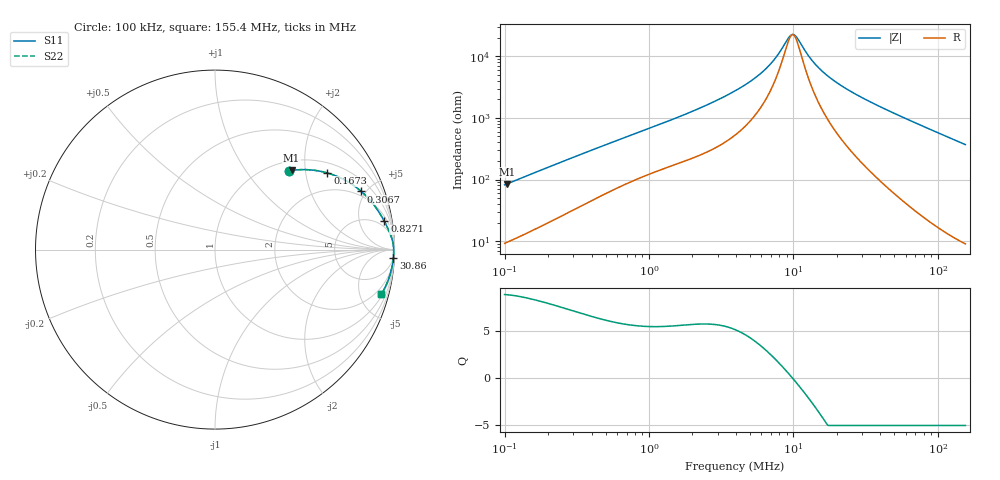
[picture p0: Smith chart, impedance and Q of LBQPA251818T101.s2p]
! LBQPA251818T101  S-PARAMETER MODEL  ( General Type )
! Model Generated by TAIYO YUDEN Corporation (http://www.ty-top.com)
! Version 1.0
! TAIYO YUDEN Control No. 191025NI43SB-FBB
! Copyright(c) 2019 TAIYO YUDEN CO.,LTD. All Rights Reserved.
! Product Description (link to TY-COMPAS)
! https://ds.yuden.co.jp/TYCOMPAS/or/detail?pn=LBQPA251818T101K&u=M
! Products Name : Inductors
! Characteristics :
!  Inductance : 100 uH , SRF(min) : 9.0 MHz , DC Resistance(max) : 4.81 Ohm
!  Rated Current : Saturation :160 mA , Temp Rise : 125 mA (20 degC)
!  Case Size : 2.5 x 1.8 / 0.098 x 0.071 [mm/inch] , Thickness : 1.8 / 0.071 [mm/inch]
!  (Conditions: Temperature = 25 degC , DC Bias Current/Voltage = 0A / 0V)
! External Node Assignments :
!  1  o---GGG---o  2
! GND o---------o GND
! Frequency Range : 0.1MHz  -  155.401204MHz  [ 402 STEP ]
# MHz S RI R 50
! Freq[MHz].  S11 Real  S11 Imag  S21 Real  S21 Imag  S12 Real  S12 Imag  S22 Real  S22 Imag
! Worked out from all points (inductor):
!   401 points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, 100 kHz to 155.4 MHz, reference 50 ohm
!   read as one part in series: L = 128 uH near 103.7 kHz
!   highest Q = 8.83 at 103.7 kHz (marker M1), where L = 129 uH
!   self-resonance near 9.698 MHz
!   S11 on the Smith chart (normalised r, x): 100 kHz: 1.18, +1.63; 167.3 kHz: 1.32, +2.65; 306.7 kHz: 1.66, +4.65; 827.1 kHz: 3, +11; 30.86 MHz: 4, -41; 155.4 MHz: 1.18, -7.37
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0.1  0.4112 0.4388  0.5888 -0.4388  0.5888 -0.4388  0.4112 0.4388
0.103743  0.4267 0.4412  0.5733 -0.4412  0.5733 -0.4412  0.4267 0.4412
0.167264  0.6261 0.4269  0.3739 -0.4269  0.3739 -0.4269  0.6261 0.4269
0.306688  0.8147 0.3242  0.1853 -0.3242  0.1853 -0.3242  0.8147 0.3242
0.342427  0.8382 0.3024  0.1618 -0.3024  0.1618 -0.3024  0.8382 0.3024
0.827072  0.9435 0.1576  0.0565 -0.1576  0.0565 -0.1576  0.9435 0.1576
1.172566  0.9627 0.119  0.0373 -0.119  0.0373 -0.119  0.9627 0.119
2.356814  0.9847 0.0633  0.0153 -0.0633  0.0153 -0.0633  0.9847 0.0633
3.942096  0.9919 0.0352  0.00815 -0.0352  0.00815 -0.0352  0.9919 0.0352
5.192861  0.9938 0.0233  0.00623 -0.0233  0.00623 -0.0233  0.9938 0.0233
6.473667  0.9947 0.0148  0.00528 -0.0148  0.00528 -0.0148  0.9947 0.0148
7.498587  0.9951 0.00951  0.00486 -0.00951  0.00486 -0.00951  0.9951 0.00951
9.177924  0.9955 0.00251  0.00448 -0.00251  0.00448 -0.00251  0.9955 0.00251
9.697959  0.9956 0.000628  0.00441 -0.000628  0.00441 -0.000628  0.9956 0.000628
10.06092  0.9956 -0.000629  0.00438 0.000629  0.00438 0.000629  0.9956 -0.000629
10.63099  0.9957 -0.00252  0.00433 0.00252  0.00433 0.00252  0.9957 -0.00252
13.49882  0.9957 -0.0109  0.00428 0.0109  0.00428 0.0109  0.9957 -0.0109
15.63597  0.9956 -0.0163  0.00437 0.0163  0.00437 0.0163  0.9956 -0.0163
18.78933  0.9954 -0.0236  0.00461 0.0236  0.00461 0.0236  0.9954 -0.0236
30.85563  0.9937 -0.048  0.00634 0.048  0.00634 0.048  0.9937 -0.048
46.22367  0.99 -0.0762  0.00999 0.0762  0.00999 0.0762  0.99 -0.0762
155.4012  0.9262 -0.2496  0.0738 0.2496  0.0738 0.2496  0.9262 -0.2496
